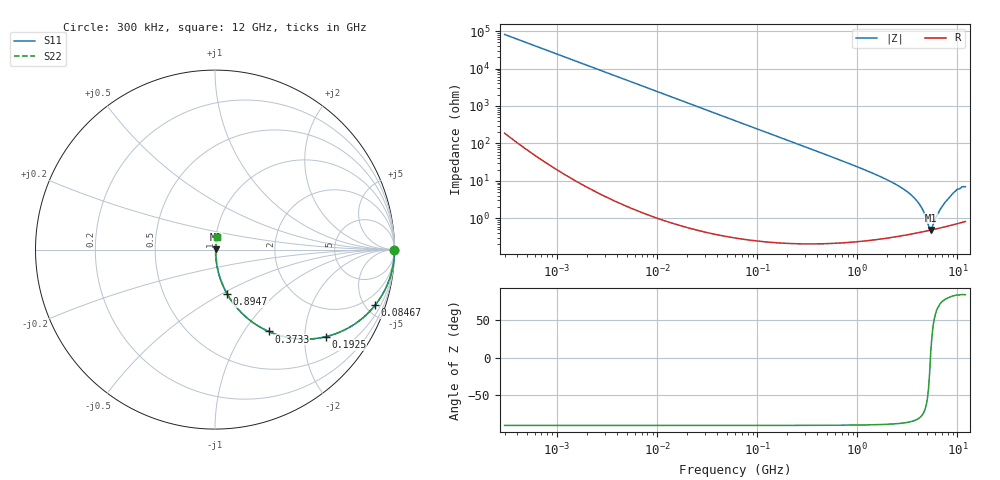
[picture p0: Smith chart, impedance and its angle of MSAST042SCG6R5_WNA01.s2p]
! MSAST042SCG6R5_WNA01  S-PARAMETER MODEL  ( General Type )
! Model Generated by TAIYO YUDEN Corporation (http://www.ty-top.com)
! Version 1.0
! TAIYO YUDEN Control No. 150820
! Copyright(c) 2015 TAIYO YUDEN CO.,LTD. All Rights Reserved.
! Product Description (link to TY-COMPAS)
! https://ds.yuden.co.jp/TYCOMPAS/or/detail?pn=MSAST042SCG6R5BWNA01&u=M
! Products Name : Multilayer Ceramic Capacitors
! Characteristics :
!  Capacitance : 6.5 pF , Rated Voltage : 25V , TCC : CG / C0G
!  Case Size : 0.4 x 0.2 / 0.016 x 0.008 [mm/inch] , Thickness : 0.2 / 0.008 [mm/inch]
!  (Conditions: Temperature = 25 degC , DC Bias Current/Voltage = 0A / 0V)
! External Node Assignments :
!  1  o---| |---o  2
! GND o---------o GND
! Frequency Range : 0.3MHz  -  12000MHz  [ 401 STEP ]
# MHz S RI R 50
! Freq[MHz].  S11 Real  S11 Imag  S21 Real  S21 Imag  S12 Real  S12 Imag  S22 Real  S22 Imag
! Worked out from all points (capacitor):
!   401 points, 300 kHz to 12 GHz, reference 50 ohm
!   read as one part in series: C = 6.51 pF near 316.3 kHz
!   lowest |Z| = 487 mohm at 5.42 GHz (marker M1)
!   series resonance near 5.375 GHz, so ESL is about 130 pH
!   S11 on the Smith chart (normalised r, x): 300 kHz: open; 84.67 MHz: 1.01, -5.77; 192.5 MHz: 1.00, -2.54; 373.3 MHz: 1.00, -1.30; 894.7 MHz: 1.00, -0.53; 12 GHz: 1.02, +0.14
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0.3  1 -0.00123  4.32e-06 0.00123  4.32e-06 0.00123  1 -0.00123
1.769972  0.9999 -0.00724  5.66e-05 0.00724  5.66e-05 0.00724  0.9999 -0.00724
10.44266  0.9982 -0.0426  0.00184 0.0426  0.00184 0.0426  0.9982 -0.0426
27.10171  0.9878 -0.1095  0.0122 0.1095  0.0122 0.1095  0.9878 -0.1095
60  0.9431 -0.2314  0.0569 0.2314  0.0569 0.2314  0.9431 -0.2314
84.66778  0.8927 -0.3091  0.1073 0.3091  0.1073 0.3091  0.8927 -0.3091
192.4766  0.6167 -0.4854  0.3833 0.4854  0.3833 0.4854  0.6167 -0.4854
353.9943  0.3216 -0.4656  0.6784 0.4656  0.6784 0.4656  0.3216 -0.4656
373.2558  0.2989 -0.4562  0.7011 0.4562  0.7011 0.4562  0.2989 -0.4562
570.2811  0.1536 -0.3581  0.8464 0.3581  0.8464 0.3581  0.1536 -0.3581
894.6982  0.0678 -0.2472  0.9322 0.2472  0.9322 0.2472  0.0678 -0.2472
2088.533  0.0127 -0.0979  0.9873 0.0979  0.9873 0.0979  0.0127 -0.0979
3026.31  0.00652 -0.0546  0.9935 0.0546  0.9935 0.0546  0.00652 -0.0546
3841.137  0.00491 -0.0309  0.9951 0.0309  0.9951 0.0309  0.00491 -0.0309
4385.161  0.00459 -0.0185  0.9954 0.0185  0.9954 0.0185  0.00459 -0.0185
5140.631  0.00466 -0.00403  0.9953 0.00403  0.9953 0.00403  0.00466 -0.00403
5420.343  0.00479 0.000763  0.9952 -0.000763  0.9952 -0.000763  0.00479 0.000763
5715.274  0.00496 0.00453  0.995 -0.00453  0.995 -0.00453  0.00496 0.00453
6699.894  0.0057 0.016  0.9943 -0.016  0.9943 -0.016  0.0057 0.016
7854.144  0.0069 0.0293  0.9931 -0.0293  0.9931 -0.0293  0.0069 0.0293
9708.23  0.00993 0.0543  0.9901 -0.0543  0.9901 -0.0543  0.00993 0.0543
12000  0.0127 0.0677  0.9873 -0.0677  0.9873 -0.0677  0.0127 0.0677
